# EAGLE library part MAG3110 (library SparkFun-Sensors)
Freescale MAG3110 3-Axis Digital (I2C) Magnetometer Freescale’s MAG3110 is a small, low-power, digital 3-axis magnetometer. The device can be used in conjunction with a 3-axis accelerometer to produce orientation independent accurate compass heading information. It features a standard I2C serial interface output and smart embedded functions. Datasheet SparkFun Products SparkFun Triple Axis Magnetometer Breakout - MAG3110 (SEN-12670)
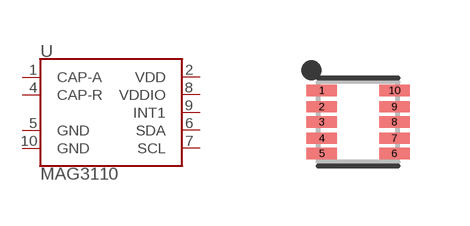
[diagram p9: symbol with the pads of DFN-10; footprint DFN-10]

Designator prefix U

## MAG3110 (PROD_ID: IC-10404)  [DFN-10]
1  CAP-A
2  VDD
4  CAP-R
5  GND
6  SDA
7  SCL
8  VDDIO
9  INT1
10  GND

## Footprint DFN-10 (pad centres in mm)
10-pin Dual-Flat No-Lead (DFN) (2.0 x 2.0 mm) (1:1 footprint) Datasheet Specifications: Pin Count: 10 Dimensions: 2.0 x 2.0 x 0.85 mm Pitch: 0.4 mm Devices Using: MAG3110
smd 0.762 x 0.279: 1 -0.91,0.787; 2 -0.91,0.381; 3 -0.91,0; 4 -0.91,-0.406; 5 -0.91,-0.787; 6 0.91,-0.787; 7 0.91,-0.406; 8 0.91,0; 9 0.91,0.381; 10 0.91,0.787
